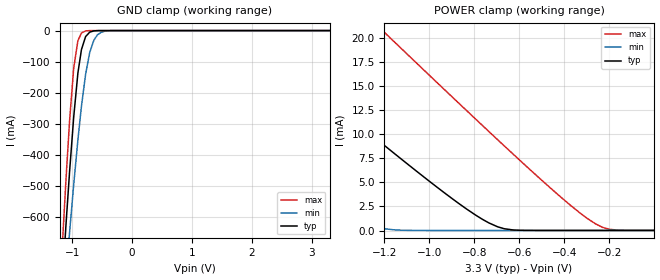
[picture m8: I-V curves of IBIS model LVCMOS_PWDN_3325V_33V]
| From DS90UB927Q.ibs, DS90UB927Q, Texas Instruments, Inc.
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|   Model
[Model] LVCMOS_PWDN_3325V_33V
Model_type Input
Vinh = 2.0V
Vinl = 0.8V
C_comp   6.98pF   6.05pF   8.06pF
[Voltage Range]   3.3V   2.97V   3.63V
[Temperature Range]   25.0   130.0   -40.0
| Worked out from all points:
|   GND clamp passes 1 mA (typ) near -0.64 V on its own axis
|   POWER clamp passes 1 mA (typ) near -0.75 V on its own axis
[GND Clamp]
-3.3V     -7.729A    -6.4A      -8.836A
-1.171V   -833.9mA   -960.8mA   -719.2mA
-1.102V   -623.3mA   -790.6mA   -477.4mA
-1.043V   -454.3mA   -650.1mA   -290.9mA
-973.5mV  -277.4mA   -494.8mA   -119.9mA
-904.2mV  -136.9mA   -352.1mA   -32.51mA
-844.8mV  -61.18mA   -243.7mA   -7.894mA
-775.5mV  -19.32mA   -140.4mA   -1.007mA
-706.2mV  -4.956mA   -70.01mA   -77.4uA
-636.9mV  -978.5uA   -30.5mA    -12.69uA
-438.9mV  -9.002uA   -1.422mA   -6.836uA
3.293V    6.997uA    0A         13.56uA
[POWER Clamp]
-3.3V     49.93mA    32.15mA    67.99mA
-2.597V   36.04mA    20.71mA    52.05mA
-1.835V   21.07mA    8.535mA    34.82mA
-1.795V   20.3mA     7.919mA    33.92mA
-1.399V   12.62mA    2.098mA    25.01mA
-1.201V   8.848mA    193.6uA    20.58mA
-864.6mV  2.724mA    4.381uA    13.1mA
-696.3mV  380uA      4.135uA    9.406mA
-399.3mV  7.606uA    3.796uA    3.128mA
-260.7mV  7.361uA    3.668uA    674uA
-201.3mV  7.269uA    3.618uA    127.6uA
-3.3mV    7.008uA    3.477uA    14.34uA
